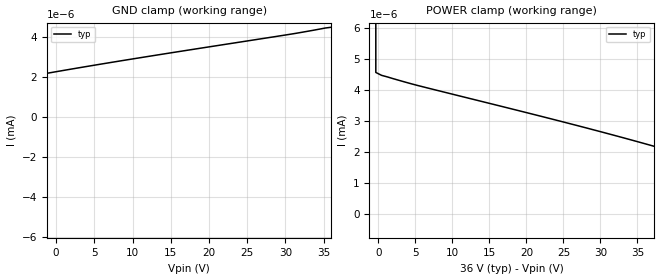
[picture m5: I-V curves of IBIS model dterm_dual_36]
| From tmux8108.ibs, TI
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| dterm_dual_36
[Model]   dterm_dual_36
Model_type   Terminator
|   typ   min   max
C_comp   6.362683e-12   NA   NA
[Voltage Range]   36   NA   NA
[Temperature Range]   27   NA   NA
[Power Clamp Reference]   36   NA   NA
[GND Clamp Reference]   0   NA   NA
[GND Clamp]
|   Voltage   I(typ)   I(min)   I(max)
-41V      -4.512A    NA         NA
-36.33V   -6.477nA   NA         NA
-35.56V   -524.1pA   NA         NA
-30.89V   -218.2pA   NA         NA
-16.89V   1.024nA    NA         NA
-5.222V   1.913nA    NA         NA
7.222V    2.735nA    NA         NA
36V       4.494nA    NA         NA
[POWER Clamp]
|   Voltage   I(typ)   I(min)   I(max)
-5V       1.488A     NA         NA
-1.111V   52.26mA    NA         NA
-333.3mV  4.568nA    NA         NA
444.4mV   4.474nA    NA         NA
5.111V    4.16nA     NA         NA
28.44V    2.756nA    NA         NA
40.89V    1.936nA    NA         NA
52.56V    1.052nA    NA         NA
66.56V    -191.3pA   NA         NA
68.89V    -365.2pA   NA         NA
72V       -549pA     NA         NA
